PROGRAM MAIN
VAR
	aComboboxEntries : ARRAY [1..5] OF ST_ComboboxEntry;
	aTexts : ARRAY [1..5] OF STRING := ['Text 1','Text 2','Text 3','Text 4','Text 5'];
	bIni: BOOL := TRUE;
	nCounter: INT;
END_VAR

// set the Combobox entries in the first cycle
IF bIni THEN
	FOR nCounter := 1 TO 5 DO
		aComboboxEntries[nCounter].id := nCounter;
		aComboboxEntries[nCounter].text := CONCAT('Array entry ', INT_TO_STRING(nCounter));
		aComboboxEntries[nCounter].value := nCounter * 10;
	END_FOR
	
	bIni := FALSE;
END_IF

END_PROGRAM
